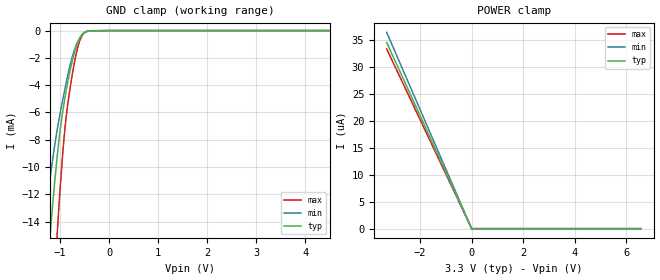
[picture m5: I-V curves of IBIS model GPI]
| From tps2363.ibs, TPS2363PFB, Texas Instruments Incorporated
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|   GPI MODEL
[Model]   GPI
Model_type   Input
|   Valid for GPIA1/B1, GPIA2/B2
Vinl = 0.8V
Vinh = 2.0V
|   typ   min   max
C_comp   2.567pF   2.702pF   2.441pF
[Voltage Range]   3.300V   3.000V   3.600V
|Junction Temperature
[Temperature Range]   40.0   125.0   -40.0
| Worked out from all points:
|   GND clamp passes 1 mA (typ) near -0.65 V on its own axis
[GND Clamp]
|   Voltage   I(typ)   I(min)   I(max)
-3.3V     -183.6mA   -124.8mA   -260mA
-1.34V    -21.7mA    -15.02mA   -35.4mA
-1.191V   -14.46mA   -10.51mA   -23.68mA
-1.063V   -9.351mA   -7.349mA   -15.12mA
-1.053V   -9.011mA   -7.137mA   -14.53mA
-973.5mV  -6.6mA     -5.563mA   -10.28mA
-914.1mV  -5.183mA   -4.471mA   -7.668mA
-815.1mV  -3.253mA   -2.815mA   -4.666mA
-716.1mV  -1.713mA   -1.503mA   -2.501mA
-617.1mV  -668.5uA   -641.6uA   -935.5uA
-468.6mV  -71uA      -96.01uA   -76.4uA
6.58V     0A         0A         0A
[POWER Clamp]
|   Voltage   I(typ)   I(min)   I(max)
-3.3V     34.48uA    36.35uA    33.28uA
-3.29V    34.34uA    36.21uA    33.15uA
0V        0A         0A         0A
6.58V     0A         0A         0A
